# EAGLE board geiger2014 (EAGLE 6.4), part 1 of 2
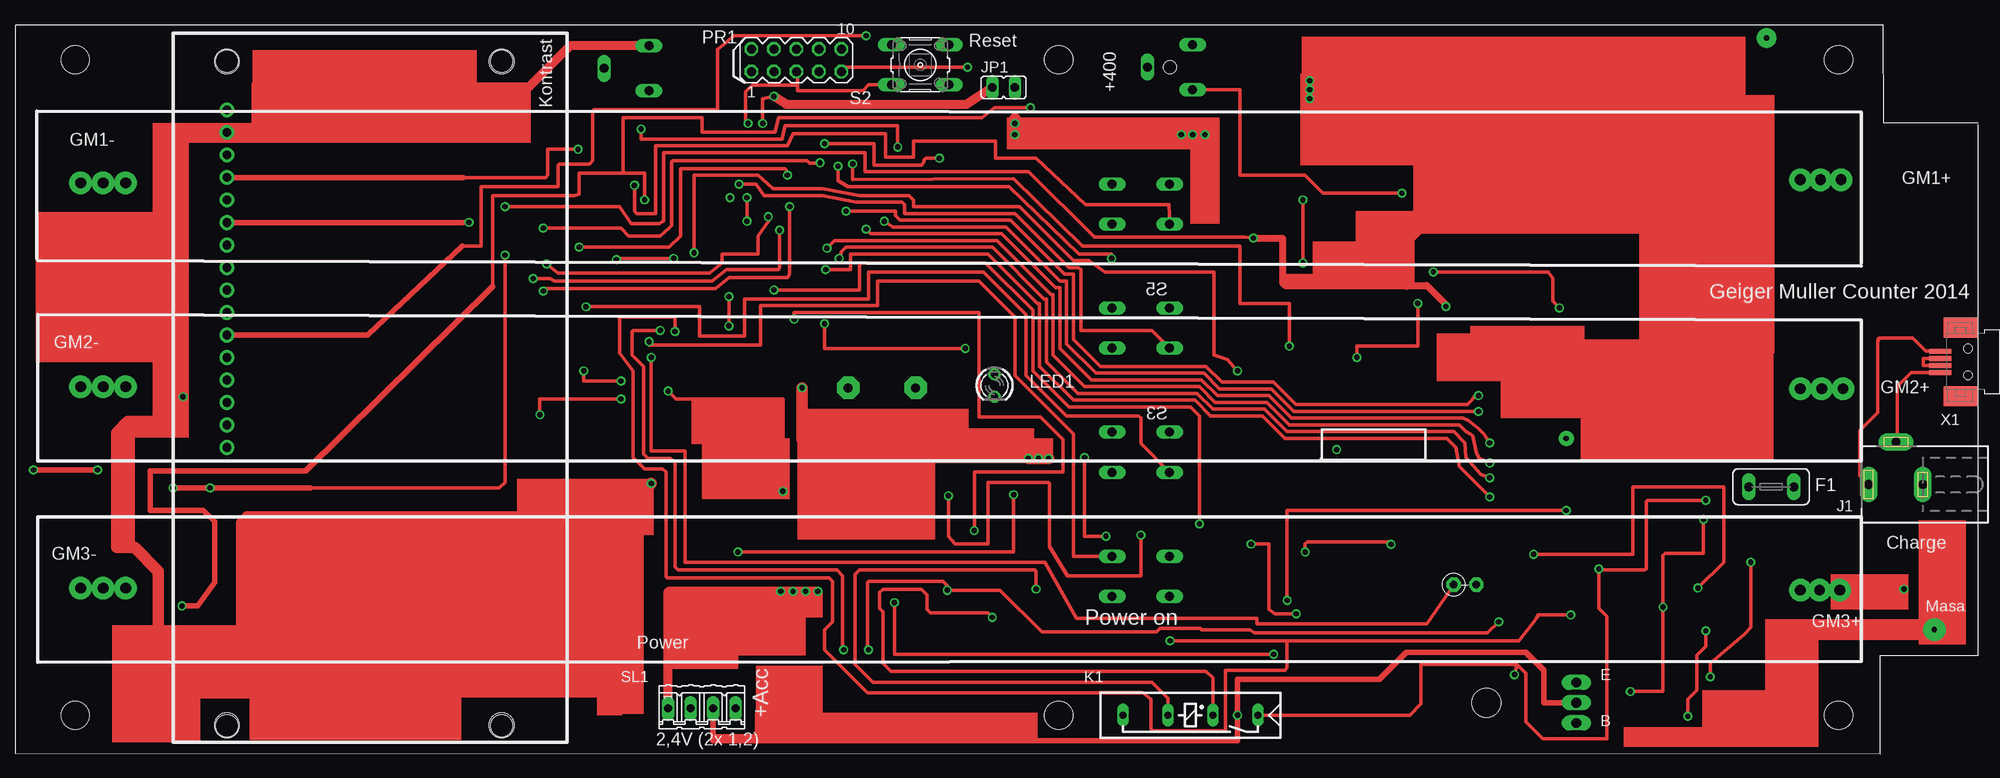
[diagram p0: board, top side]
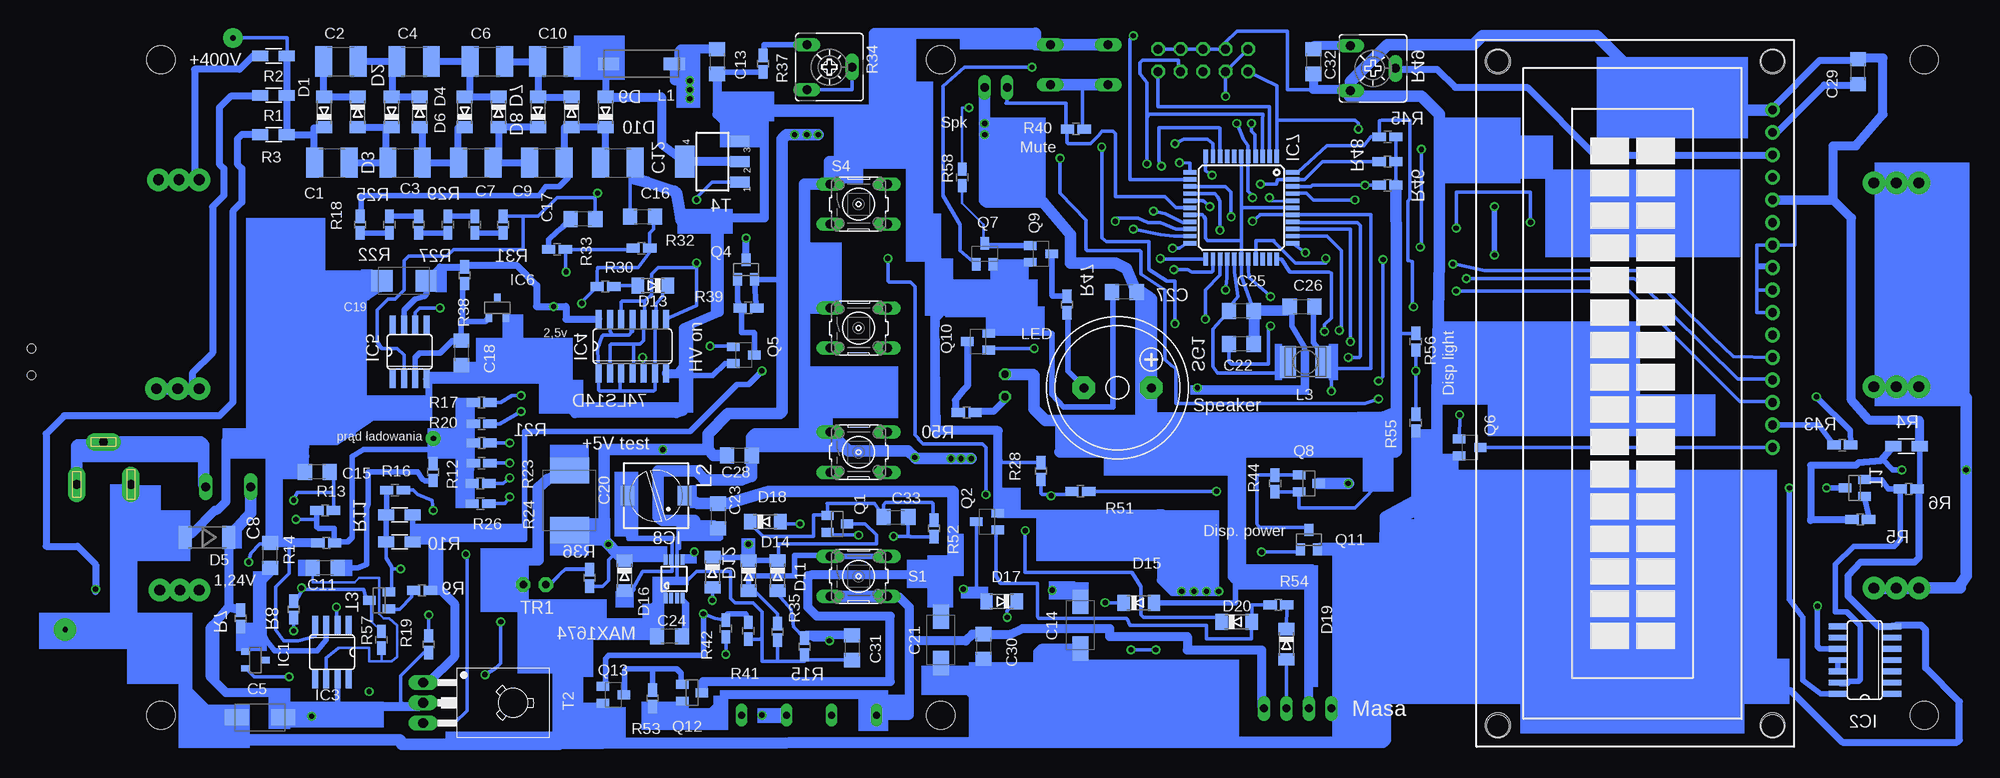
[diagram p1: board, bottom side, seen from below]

No outline drawn. Coordinates in mm, seen from the top.
Copper layers (1*16): Top 0.035mm / dielectric 1.5mm / Bottom 0.035mm
Design rules "default *": minimum track width 10mil, minimum drill 24mil, track to track 5mil, track to pad 5mil, pad to pad 5mil, via to via 5mil, smd to smd 5mil, copper to edge 40mil, drill to drill 8mil, minimum pad ring 10mil, minimum via ring 8mil, stop-mask expansion 4mil, vias tented up to drill 0mil, thermal gap 10mil
Holes 3.2 mm at 6.74,4.3 117.74,4.3 205.74,4.3 205.74,78.3 117.74,78.3 6.74,78.3
Holes 2.8 mm at 54.86,3.17 23.88,3.17 23.88,78.11 54.86,78.11
Holes 1.5 mm at 130.3,77.47

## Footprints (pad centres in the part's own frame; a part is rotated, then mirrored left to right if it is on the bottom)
C1812 = smd 1.9 x 3.4: 1 -1.95,0; 2 1.95,0
C/6032-28W = smd 2.75 x 1.8: + 2.625,0; - -2.625,0
C1206 = smd 1.6 x 1.8: 1 -1.4,0; 2 1.4,0
SMC_C = smd 2.4 x 2.4: + -2.5,0; - 2.5,0
E/7260-38W = smd 2.95 x 4.4: + 3.375,0; - -3.375,0
MINIMELF = smd 1.4 x 1.8: A 1.7,0; C -1.7,0
SOD87 = smd 1.45 x 2.6: 1 -2.445,0; 2 2.445,0
TUXGR_16X2_R2 = drill 1 pad 1.676: 1 -32,15.5; 2 -29.46,15.5; 3 -26.92,15.5; 4 -24.38,15.5; 5 -21.84,15.5; 6 -19.3,15.5; 7 -16.76,15.5; 8 -14.22,15.5; 9 -11.68,15.5; 10 -9.14,15.5; 11 -6.6,15.5; 12 -4.06,15.5; 13 -1.52,15.5; 14 1.02,15.5; 15 3.56,15.5; 16 6.1,15.5 | hole 2.5: -37.5,-15.5; 37.5,-15.5; -37.5,15.5; 37.5,15.5
TE5 = drill 1.016 long: 1 -2.54,0; 2 2.54,0
DBZ_R-PDSO-G3 = smd 0.7 x 1: 1 -0.95,-1.1; 2 0.95,-1.1; 3 0,1.1
SO14 = smd 0.66 x 2.032: 1 -3.81,-3.073; 2 -2.54,-3.073; 3 -1.27,-3.073; 4 0,-3.073; 5 1.27,-3.073; 6 2.54,-3.073; 7 3.81,-3.073; 8 3.81,3.073; 9 2.54,3.073; 10 1.27,3.073; 11 0,3.073; 12 -1.27,3.073; 13 -2.54,3.073; 14 -3.81,3.073
SO08 = smd 0.66 x 2.032: 1 -1.905,-3.073; 2 -0.635,-3.073; 3 0.635,-3.073; 4 1.905,-3.073; 5 1.905,3.073; 6 0.635,3.073; 7 -0.635,3.073; 8 -1.905,3.073
TQFP44 = smd 1.5 x 0.5: 1 -5.8,4; 2 -5.8,3.2; 3 -5.8,2.4; 4 -5.8,1.6; 5 -5.8,0.8; 6 -5.8,0; 7 -5.8,-0.8; 8 -5.8,-1.6; 9 -5.8,-2.4; 10 -5.8,-3.2; 11 -5.8,-4; 23 5.8,-4; 24 5.8,-3.2; 25 5.8,-2.4; 26 5.8,-1.6; 27 5.8,-0.8; 28 5.8,0; 29 5.8,0.8; 30 5.8,1.6; 31 5.8,2.4; 32 5.8,3.2; 33 5.8,4 | smd 0.5 x 1.5: 12 -4,-5.8; 13 -3.2,-5.8; 14 -2.4,-5.8; 15 -1.6,-5.8; 16 -0.8,-5.8; 17 0,-5.8; 18 0.8,-5.8; 19 1.6,-5.8; 20 2.4,-5.8; 21 3.2,-5.8; 22 4,-5.8; 34 4,5.8; 35 3.2,5.8; 36 2.4,5.8; 37 1.6,5.8; 38 0.8,5.8; 39 0,5.8; 40 -0.8,5.8; 41 -1.6,5.8; 42 -2.4,5.8; 43 -3.2,5.8; 44 -4,5.8
UMAX8 = smd 0.45 x 1.2: 1 -0.975,-2.175; 2 -0.325,-2.175; 3 0.325,-2.175; 4 0.975,-2.175; 5 0.975,2.175; 6 0.325,2.175; 7 -0.325,2.175; 8 -0.975,2.175
DCJ0303 = drill 1 pad 2 long: 1 0,3.1; 2 4.8,0; 3 0,-3
JP1 = drill 0.914 long: 1 0,-1.27; 2 0,1.27
REED = drill 0.813 long: 1 -17.78,2.54; 3 -12.7,2.54; 5 -7.62,2.54; 7 -2.54,2.54
L8530M = smd 2.4 x 1.4: 1 -3.7,0; 2 3.7,0
PIS2816 = smd 2.2 x 1.6: 1 0,3.2; 2 0,-3.2
L4532P = smd 1.8 x 3.6: 1 -2,0; 2 2,0
LED3MM = drill 0.813 octagon: A -1.27,0; K 1.27,0
MA05-2 = drill 1.016 octagon: 1 -5.08,-1.27; 2 -5.08,1.27; 3 -2.54,-1.27; 4 -2.54,1.27; 5 0,-1.27; 6 0,1.27; 7 2.54,-1.27; 8 2.54,1.27; 9 5.08,-1.27; 10 5.08,1.27
SOT23 = smd 1 x 1.4: 1 -0.95,-1.1; 2 0.95,-1.1; 3 0,1.1
SC59-BEC = smd 1 x 1.4: B -0.95,-1.2; C 0,1.2; E 0.95,-1.2
R1206W = smd 1.8 x 1.2: 1 -1.499,0; 2 1.499,0
R0805W = smd 1.5 x 1: 1 -0.94,0; 2 0.94,0
CA6V = drill 1.016 long: A -2.54,-2.54; E 2.54,-2.54; S 0,2.54
B3F-10XX = drill 1.016 long: 1 -3.251,2.261; 2 3.251,2.261; 3 -3.251,-2.261; 4 3.251,-2.261
F/HMB = drill 1.016 pad 2.54 octagon: + 3.81,0; - -3.81,0
04P = drill 0.914 long: 1 -3.81,0; 2 -1.27,0; 3 1.27,0; 4 3.81,0
TO126 = drill 1.118 long: 1 -2.286,-5.08; 2 0,-5.08; 3 2.286,-5.08 | hole 3.302: 0,5.08
SOT223 = smd 1.219 x 2.235: 1 -2.311,-3.099; 2 0,-3.099; 3 2.311,-3.099 | smd 3.6 x 2.2: 4 0,3.099
RS-2,5 = drill 0.813 pad 1.6 octagon: 1 -1.27,0; 2 1.27,0
32005-00X = smd 2.5 x 0.55: 1 3.15,1.2; 2 3.15,0.4; 3 3.15,-0.4; 4 3.15,-1.2 | smd 3.8 x 2.25: M1 0.85,3.875; M2 0.85,-3.875 | hole 1: 0,1.5; 0,-1.5

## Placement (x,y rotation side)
C1  [C1812]  186.44,66.67 0 bottom
C2  [C1812]  185.42,78.11 0 bottom
C3  [C1812]  178.18,66.67 0 bottom
C4  [C1812]  177.16,78.11 0 bottom
C5  [C/6032-28W]  194.56,4.06 0 bottom
C6  [C1812]  168.91,78.11 0 bottom
C7  [C1812]  170.18,66.67 0 bottom
C8  [C1206]  193.42,22.35 90 bottom
C9  [C1812]  162.18,66.67 0 bottom
C10  [C1812]  161.29,78.11 0 bottom
C11  [C1206]  187.2,20.95 180 bottom
C12  [C1812]  154.18,66.67 0 bottom
C13  [C1206]  143,78.11 270 bottom
C14  [C/6032-28W]  101.98,14.48 90 bottom
C15  [C1206]  188.09,31.75 180 bottom
C16  [C1206]  151.38,60.58 0 bottom
C17  [C1206]  158.12,60.33 180 bottom
C18  [C1206]  171.83,45.21 270 bottom
C19  [SMC_C]  178.31,53.34 180 bottom
C20  [E/7260-38W]  159.64,28.57 270 bottom
C21  [C/6032-28W]  117.73,12.83 90 bottom
C22  [C1206]  83.82,46.23 180 bottom
C23  [C1206]  142.88,26.8 270 bottom
C24  [C1206]  148.34,13.21 180 bottom
C25  [C1206]  83.82,49.91 180 bottom
C26  [C1206]  76.96,50.42 0 bottom
C27  [C1206]  97.03,52.07 180 bottom
C28  [C1206]  140.46,33.66 180 bottom
C29  [C1206]  14.22,76.96 90 bottom
C30  [C1206]  112.9,12.06 270 bottom
C31  [C1206]  127.76,11.94 270 bottom
C32  [C1206]  75.69,78.11 270 bottom
C33  [C1206]  122.81,26.67 0 bottom
D1  [MINIMELF]  187.32,72.39 90 bottom
D2  [MINIMELF]  183.51,72.39 270 bottom
D3  [MINIMELF]  179.71,72.39 90 bottom
D4  [MINIMELF]  176.53,72.39 270 bottom
D5  [SOD87]  200.53,24.38 180 bottom
D6  [MINIMELF]  171.45,72.39 90 bottom
D7  [MINIMELF]  167.64,72.39 270 bottom
D8  [MINIMELF]  163.19,72.39 90 bottom
D9  [MINIMELF]  159.38,72.39 270 bottom
D10  [MINIMELF]  155.57,72.39 90 bottom
D11  [MINIMELF]  136.14,20.07 270 bottom
D12  [MINIMELF]  143.51,20.45 270 bottom
D13  [MINIMELF]  150.24,52.83 180 bottom
D14  [MINIMELF]  139.45,20.07 270 bottom
D15  [MINIMELF]  95.38,17.02 0 bottom
D16  [MINIMELF]  153.42,20.07 270 bottom
D17  [MINIMELF]  110.87,17.14 180 bottom
D18  [MINIMELF]  137.54,26.16 0 bottom
D19  [MINIMELF]  78.74,12.32 270 bottom
D20  [MINIMELF]  84.33,14.86 0 bottom
DIS1  TUXGR_16X2_R2  [TUXGR_16X2_R2]  39.37,40.64 270 bottom
F1  [TE5]  198.12,30.1 0 top
IC1  LM4041A12DBZ  [DBZ_R-PDSO-G3]  195.07,10.54 270 bottom
IC2  74LS14D  [SO14]  13.46,10.54 90 bottom
IC3  MAX4105ESA  [SO08]  186.44,11.43 180 bottom
IC4  74LS14D  [SO14]  152.53,45.97 0 bottom
IC5  MAX4105ESA  [SO08]  177.67,45.34 0 bottom
IC6  LM4041A12DBZ  [DBZ_R-PDSO-G3]  167.77,50.29 0 bottom
IC7  MEGA16-A  [TQFP44]  83.82,61.59 270 bottom
IC8  MAX1674  [UMAX8]  147.83,19.68 0 bottom
J1  [DCJ0303]  212.22,30.35 90 top
JP1  [JP1]  111.51,75.18 270 top
K1  35701331  [REED]  122.43,6.86 180 top
L1  [L8530M]  151.51,77.85 0 bottom
L2  [PIS2816]  149.86,29.08 270 bottom
L3  [L4532P]  76.58,44.2 180 bottom
LED1  [LED3MM]  110.49,41.53 270 top
PR1  [MA05-2]  88.14,78.23 0 top
Q1  BSS123  [SOT23]  129.41,25.91 270 bottom
Q2  MUN2212T1  [SC59-BEC]  112.52,26.16 90 bottom
Q4  BSS84  [SOT23]  139.7,54.61 0 bottom
Q5  MUN2212T1  [SC59-BEC]  139.95,44.96 270 bottom
Q6  MUN2212T1  [SC59-BEC]  58.04,34.54 270 bottom
Q7  MUN2212T1  [SC59-BEC]  112.78,56.39 0 bottom
Q8  BSS84  [SOT23]  76.2,30.48 270 bottom
Q9  MUN2212T1  [SC59-BEC]  106.43,56.39 270 bottom
Q10  MUN2212T1  [SC59-BEC]  113.54,46.48 90 bottom
Q11  BSS123  [SOT23]  76.2,24.13 0 bottom
Q12  BSS84  [SOT23]  145.8,6.86 270 bottom
Q13  MUN2212T1  [SC59-BEC]  154.69,6.6 270 bottom
R1  [R1206W]  193.04,74.3 180 bottom
R2  [R1206W]  193.04,78.74 180 bottom
R3  [R1206W]  193.04,69.85 180 bottom
R4  [R1206W]  8.76,34.67 0 bottom
R5  [R0805W]  13.97,26.42 180 bottom
R6  [R0805W]  8.51,29.84 0 bottom
R7  [R0805W]  196.72,15.24 90 bottom
R8  [R0805W]  190.75,16.26 270 bottom
R9  [R0805W]  176.28,18.41 180 bottom
R10  [R1206W]  178.82,23.88 180 bottom
R11  [R1206W]  178.82,26.92 180 bottom
R12  [R0805W]  175.01,31.75 270 bottom
R13  [R0805W]  187.2,27.43 0 bottom
R14  [R0805W]  187.07,23.75 0 bottom
R15  [R0805W]  133.1,12.06 90 bottom
R16  [R0805W]  179.32,29.72 180 bottom
R17  [R0805W]  169.54,39.62 180 bottom
R18  [R0805W]  183.26,59.69 90 bottom
R19  [R0805W]  175.51,12.32 270 bottom
R20  [R0805W]  169.54,37.21 180 bottom
R21  [R0805W]  169.54,35.05 180 bottom
R22  [R0805W]  179.96,59.69 270 bottom
R23  [R0805W]  169.54,32.77 180 bottom
R24  [R0805W]  169.67,30.48 180 bottom
R25  [R0805W]  176.66,59.69 90 bottom
R26  [R0805W]  169.67,28.19 180 bottom
R27  [R0805W]  173.35,59.69 270 bottom
R28  [R0805W]  106.43,31.88 90 bottom
R29  [R0805W]  170.31,59.69 90 bottom
R30  [R0805W]  155.57,52.7 0 bottom
R31  [R0805W]  167.13,59.69 270 bottom
R32  [R0805W]  151.51,57.02 0 bottom
R33  [R0805W]  161.04,56.9 180 bottom
R34  [CA6V]  130.3,77.47 270 bottom
R35  [R0805W]  136.14,13.72 270 bottom
R36  [R0805W]  157.35,19.81 270 bottom
R37  [R0805W]  137.79,77.85 270 bottom
R38  [R0805W]  171.45,53.98 270 bottom
R39  [R0805W]  139.45,50.29 180 bottom
R40  [R0805W]  102.49,70.48 0 bottom
R41  [R0805W]  139.45,13.84 270 bottom
R42  [R0805W]  141.99,14.1 90 bottom
R43  [R0805W]  16,34.8 0 bottom
R44  [R0805W]  80.01,30.48 270 bottom
R45  [R0805W]  67.31,69.6 180 bottom
R46  [R0805W]  67.31,64.14 180 bottom
R47  [R0805W]  103.5,50.67 90 bottom
R48  [R0805W]  67.31,66.8 180 bottom
R49  [CA6V]  68.96,77.34 270 bottom
R50  [R0805W]  114.81,38.48 0 bottom
R51  [R0805W]  101.98,29.59 180 bottom
R52  [R0805W]  118.49,25.4 270 bottom
R53  [R0805W]  150.24,6.22 270 bottom
R54  [R0805W]  79.63,16.76 0 bottom
R55  [R0805W]  64.14,37.34 270 bottom
R56  [R0805W]  64.14,46.48 270 bottom
R57  [R0805W]  180.85,12.83 90 bottom
R58  [R0805W]  115.32,65.02 90 bottom
S1  [B3F-10XX]  127,20 0 bottom
S2  [B3F-10XX]  102.11,77.72 0 top
S3  [B3F-10XX]  127,34 0 bottom
S4  [B3F-10XX]  127,62 0 bottom
S5  [B3F-10XX]  127,48 0 bottom
SG1  F/HMB  [F/HMB]  97.79,41.27 0 bottom
SL1  [04P]  77.47,5.08 0 top
T1  BCX70SMD  [SOT23]  14.61,29.97 90 bottom
T2  BD139  [TO126]  171.07,5.71 270 bottom
T3  BCX70SMD  [SOT23]  181.1,17.27 90 bottom
T4  [SOT223]  143.51,66.8 90 bottom
TR1  [RS-2,5]  163.58,19.05 0 top
X1  MINI-USB_SHIELD4P-32005-00X  [32005-00X]  220.34,44.2 180 top

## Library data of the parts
C1-C33 L1-L3 = rcl
D1-D4 D6-D20 = diode
D5 = semicon-smd-ipc
DIS1 = display-lcd; OC_FARNELL: unknown; OC_NEWARK: unknown
F1 = fuse; OC_FARNELL: unknown; OC_NEWARK: unknown
IC1 IC6 = texas; MPN: LM4041A12IDBZR; OC_FARNELL: 1407949; OC_NEWARK: 58K5875
IC2 = 74xx-us
IC3 IC5 = maxim; MPN: MAX4105ESA+; OC_FARNELL: unknown; OC_NEWARK: 67K5150
IC4 = 74xx-eu
IC7 = atmel; MPN: ATMEGA16-16AU; OC_FARNELL: 9171134; OC_NEWARK: 96K6515
IC8 = maxim; MF: MAXIM; MPN: MAX1674EUA+; OC_FARNELL: 1379864; OC_NEWARK: 23K5719
J1 = con-jack; OC_FARNELL: unknown; OC_NEWARK: unknown
JP1 = jumper
K1 = relay; OC_FARNELL: unknown; OC_NEWARK: unknown
LED1 = led
PR1 = con-lstb; OC_FARNELL: unknown; OC_NEWARK: unknown
Q1 Q4 Q8 Q11 Q12 = transistor-small-signal
Q2 Q5-Q7 Q9 Q10 Q13 = transistor-npn
R1-R33 R35-R48 R50-R58 = resistor
R34 R49 = pot
S1-S5 = switch-omron; MPN: B3F-1000; OC_FARNELL: 176432; OC_NEWARK: 36M3542
SG1 = buzzer; OC_FARNELL: unknown; OC_NEWARK: unknown
SL1 = con-amp-quick; OC_FARNELL: unknown; OC_NEWARK: unknown
T1 T3 = transistor-neu-to92
T2 = transistor
T4 = zetex; OC_FARNELL: unknown; OC_NEWARK: unknown
TR1 = discrete
X1 = con-cypressindustries; OC_FARNELL: unknown; OC_NEWARK: unknown

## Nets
N$1: C13.1 C19.+ IC2.14 IC4.14 IC5.7 L1.2 Q4.3 R38.1 T1.3
N$4: F1.2 J1.2 J1.3 X1.1
N$6: R5.1 T1.1
N$7: C4.2 C6.1 D6.A D7.C
N$8: C11.2 IC3.6 R57.1
N$9: R9.2 T3.1
N$10: C11.1 R12.2
N$12: IC7.34 R9.1 R10.1 R11.1 T2.1
N$13: Q10.C R50.1
N$14: DIS1.16 Q6.C
N$15: C8.1 IC1.1 IC3.3 R7.1
N$16: IC3.2 R12.1 R13.1 R14.2 R17.2 R20.2 R21.2 R23.2 R24.2 R26.2
N$18: Q4.1 Q5.C R39.2
N$19: C30.1 K1.7 Q12.2 R53.2 S1.3 S1.4 SL1.4
N$20: IC7.1 PR1.1 Q10.B
N$22: Q12.1 Q13.C R53.1
N$24: IC7.24 R26.1
N$25: D14.A IC7.36 R35.1 S1.1 S1.2
N$26: IC7.21 R21.1
N$27: D18.A IC7.26
N$28: D17.A K1.5 Q2.C
N$29: C22.2 IC7.29
N$30: IC7.22 R23.1
N$31: D12.A R16.1
N$33: IC2.13 R6.1 T1.2
N$35: C20.+ C27.1 C28.2 D15.A D16.C IC8.5 IC8.8 JP1.2 LED1.A Q4.2 Q8.2 R36.2 R39.1 R44.2 R45.1 R46.1 R48.1 R56.1 SG1.+ SL1.2
N$36: IC7.23 R24.1
N$37: IC7.10 Q6.B
N$39: IC2.11 IC2.12
N$40: IC7.19 R17.1
N$41: C2.1 D1.A D2.C
N$42: R4.1 R5.2
N$43: C2.2 C4.1 D3.A D4.C
N$44: R1.2
N$45: R2.2
N$46: R3.2
N$47: C10.2 D10.A L1.1 T4.2 T4.4
N$48: R18.1 R22.2
N$49: C1.2 C3.1 D2.A D3.C
N$50: C1.1 D1.C R1.1 R2.1 R3.1
N$51: IC4.2 IC4.4 IC4.8 IC4.10 IC4.12 T4.1
N$52: R22.1 R25.2
N$53: C3.2 C7.1 D4.A D6.C
N$54: R47.1 SG1.-
N$55: R25.1 R27.2
N$56: C7.2 C9.1 D7.A D8.C
N$57: R27.1 R29.2
N$58: C6.2 C10.1 D8.A D9.C
N$59: C9.2 C12.1 D9.A D10.C R18.2
N$60: IC2.10 IC7.41 R58.2
N$61: R29.1 R31.2
N$62: C17.1 IC5.2 R31.1 R34.E R34.S
N$63: C33.1 D18.C Q1.1 R52.1
N$64: D13.C IC4.1 IC4.3 IC4.6 IC4.9 IC4.11 IC4.13
N$65: D13.A R30.2
N$66: C16.2 IC4.5 R30.1 R32.2
N$67: Q9.C R47.2
N$69: C18.1 IC5.3 IC6.1 R38.2
N$71: D15.C R42.1
N$72: IC5.6 R32.1 R33.1
N$73: D20.A Q2.B R54.1
N$74: C17.2 R33.2
N$76: R34.A R37.1
N$77: D16.A IC8.7 L2.2
N$79: C24.1 IC8.4
N$80: D20.C IC7.25
N$82: IC7.37 R36.1 TR1.1
N$84: IC7.4 PR1.5 R40.2 S2.3 S2.4
N$85: C25.2 IC7.27 L3.2
N$86: LED1.K R50.2
N$89: IC7.42 R46.2 S4.3
N$90: IC7.43 R48.2 S5.3
N$92: IC7.2 PR1.9 Q7.B
N$94: DIS1.15 R43.1
N$95: DIS1.14 IC7.16
N$96: DIS1.13 IC7.15
N$97: DIS1.3 R49.S
N$98: DIS1.12 IC7.14
N$100: DIS1.6 IC7.12
N$101: DIS1.4 IC7.11
N$102: IC7.44 R45.2 S3.3
N$104: DIS1.11 IC7.13
N$117: IC7.20 R20.1
N$119: D19.C R54.2
N$131: R8.1 R57.2 T2.3 T3.3
N$135: Q7.C Q9.B R58.1
N$136: D11.C D12.C D14.C Q1.3 Q13.B R41.1 R42.2
N$137: C5.- C8.2 C12.2 C13.2 C14.- C15.2 C16.1 C18.2 C19.- C20.- C21.- C22.1 C23.2 C24.2 C25.1 C26.1 C27.2 C28.1 C29.2 C30.2 C31.2 C32.2 C33.2 D5.2 DIS1.1 DIS1.5 DIS1.7 DIS1.8 DIS1.9 DIS1.10 IC1.2 IC2.7 IC3.4 IC4.7 IC5.4 IC6.2 IC7.6 IC7.18 IC7.28 IC7.39 IC8.1 IC8.6 J1.1 PR1.4 PR1.6 PR1.8 PR1.10 Q2.E Q5.E Q6.E Q7.E Q9.E Q10.E Q11.2 Q13.E R4.2 R6.2 R14.1 R15.1 R28.2 R35.2 R37.2 R41.2 R49.E R52.2 R55.2 S2.1 S2.2 S3.1 S4.1 S5.1 SL1.1 T4.3 TR1.2 X1.4
N$138: C14.+ C15.1 IC7.35 K1.1 R10.2 R11.2 R13.2 R16.2 T3.2
N$139: C21.+ C23.1 L2.1 Q12.3
N$140: C5.+ D5.1 D17.C D19.A F1.1 IC3.7 K1.3 R7.2 R8.2 R19.2 SL1.3 T2.2
N$141: Q1.2 R28.1 R51.2
N$142: C26.2 IC7.5 IC7.17 IC7.38 JP1.1 L3.1 PR1.2 PR1.3 R40.1 R51.1
N$143: Q8.1 Q11.3 R44.1
N$144: IC7.3 PR1.7 Q5.B
N$145: X1.2 X1.3
N$146: C31.1 D11.A IC7.33 R15.2 R19.1
N$147: IC7.9 Q11.1
N$148: IC7.30 R55.1 R56.2
N$149: C29.1 C32.1 DIS1.2 Q8.3 R43.2 R49.A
